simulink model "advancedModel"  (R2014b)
settings: Solver=ode45  StartTime=0.0  StopTime=1000  RelTol=1e-3

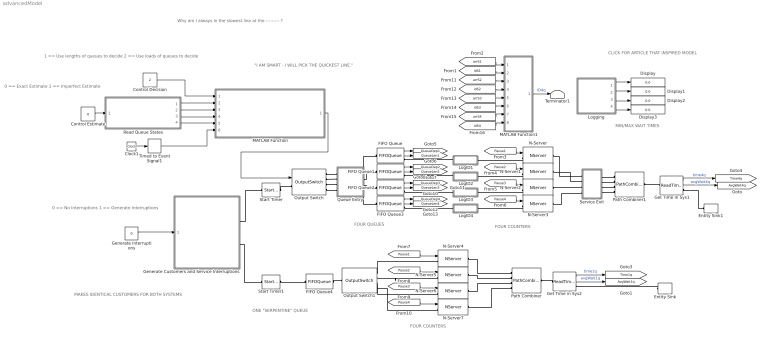
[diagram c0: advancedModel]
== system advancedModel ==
  note: 1 == Use lengths of queues to decide 2 == Use loads of queues to decide
  note: Why am I always in the slowest line at the --------- ?
  note: MAKES IDENTICAL CUSTOMERS FOR BOTH SYSTEMS
  note: "I AM SMART - I WILL PICK THE QUICKEST LINE."
  note: ONE "SERPENTINE" QUEUE
  note: FOUR COUNTERS
  note: FOUR COUNTERS
  note: FOUR QUEUES
  note: CLICK FOR ARTICLE THAT INSPIRED MODEL
  note: MIN/MAX WAIT TIMES
  note: 0 == Exact Estimate 1 == Imperfect Estimate
  note: 0 == No Interruptions 1 == Generate Interruptions
  Clock1 : Clock
  Control Decision : Constant  Value=2
  Control Estimate : Constant  Value=0
  Display{,1..3} (4 alike) : Display
  Entity Sink : EntitySink
  Entity Sink1 : EntitySink
  FIFO Queue{,1..3} (4 alike) : FIFOQueue  Capacity=inf  StatNumberDeparted=on  StatNumberInBlock=on
  FIFO Queue4 : FIFOQueue  Capacity=inf
  Generate Customers and Service Interruptions : Subsystem
  Generate Interruptions : Constant  Value=0
  Get Time In Sys1 : ReadTimer  StatTimeElapsed=on  StatAverageTimeElapsed=on
  Get Time in Sys2 : ReadTimer  TimerTag=T2  StatTimeElapsed=on  StatAverageTimeElapsed=on
  LogID1 : Subsystem
  LogID2 : Subsystem
  LogID3 : Subsystem
  LogID4 : Subsystem
  Logging : Subsystem
  MATLAB Function : MATLAB Function  TreatAsAtomicUnit=on
  MATLAB Function1 : MATLAB Function  TreatAsAtomicUnit=on
  N-Server{,1..7} (8 alike) : NServer  NumberOfServers=1  ServiceTimeFrom=Attribute  ServiceTime=sTime  AttributeName=sTime  AllowServiceControl=on
  Output Switch : OutputSwitch  NumberOutputPorts=4  SwitchingCriterion=From signal port p  InitialConditionsOpt=on
  Output Switch1 : OutputSwitch  NumberOutputPorts=4
  Path Combiner : PathCombiner  NumberInputPorts=4
  Path Combiner1 : PathCombiner  NumberInputPorts=4
  Queue Entry : Subsystem
  Read Queue States : Subsystem
  Service Exit : Subsystem
  Start Timer : StartTimer
  Start Timer1 : StartTimer  TimerTag=T2
  Terminator1 : Terminator
  Timed to Event Signal1 : TimedToEventSignal
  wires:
  Get Time In Sys1/2 -> [AvgWait4q]  "avgWait4q"
  Get Time in Sys2/2 -> [AvgWait1q]  "avgWait1q"
  [Pause1] -> N-Server/1
  [Pause2] -> N-Server1/1
  [Pause3] -> N-Server2/1
  [Pause4] -> N-Server3/1
  [Pause1] -> N-Server4/1
  [Pause2] -> N-Server5/1
  [Pause3] -> N-Server6/1
  [Pause4] -> N-Server7/1
  MATLAB Function/1(sq) -> Output Switch/1
  Get Time in Sys2/1 -> [Time1q]  "time1q"
  Get Time In Sys1/1 -> [Time4q]  "time4q"
  Logging/1(Min4q) -> Display/1
  Logging/2(Max4q) -> Display1/1
  Logging/3(Min1q) -> Display2/1
  Logging/4(Max1q) -> Display3/1
  Control Decision/1 -> MATLAB Function/1(strat)
  Generate Interruptions/1 -> Generate Customers and Service Interruptions/1(GenInterruptions)
  FIFO Queue/1 -> [QueueDep1]
  FIFO Queue/2 -> [QueueLen1]
  FIFO Queue1/1 -> [QueueDep2]
  FIFO Queue1/2 -> [QueueLen2]
  FIFO Queue2/1 -> [QueueDep3]
  FIFO Queue2/2 -> [QueueLen3]
  FIFO Queue3/1 -> [QueueDep4]
  FIFO Queue3/2 -> [QueueLen4]
  Clock1/1 -> Timed to Event Signal1/1
  Timed to Event Signal1/1 -> MATLAB Function/6(currTime)
  Read Queue States/1(queueLens) -> MATLAB Function/2(qLengths)
  Read Queue States/2(queueLoads) -> MATLAB Function/3(qLoads)
  Read Queue States/3(servStartEvents) -> MATLAB Function/4(servStartEvents)
  Read Queue States/4(servEndEvents) -> MATLAB Function/5(servEndEvents)
  [idS3] -> MATLAB Function1/6(id3)
  [idS4] -> MATLAB Function1/8(id4)
  [arrS3] -> MATLAB Function1/5(arr3)
  [idS1] -> MATLAB Function1/2(id1)
  [arrS1] -> MATLAB Function1/1(arr1)
  [arrS4] -> MATLAB Function1/7(arr4)
  [idS2] -> MATLAB Function1/4(id2)
  [arrS2] -> MATLAB Function1/3(arr2)
  MATLAB Function1/1(id) -> Terminator1/1  "ID4q"
  Control Estimate/1 -> Read Queue States/1(UnderEstimateLoad)
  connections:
  Start Timer1/RConn1 -- FIFO Queue4/LConn1
  N-Server/LConn1 -- LogID1/RConn1
  N-Server1/LConn1 -- LogID2/RConn1
  N-Server2/LConn1 -- LogID3/RConn1
  N-Server3/LConn1 -- LogID4/RConn1
  FIFO Queue4/RConn1 -- Output Switch1/LConn1
  Entity Sink/LConn1 -- Get Time in Sys2/RConn1
  Start Timer/RConn1 -- Output Switch/LConn1
  Get Time In Sys1/LConn1 -- Path Combiner1/RConn1
  Get Time in Sys2/LConn1 -- Path Combiner/RConn1
  Entity Sink1/LConn1 -- Get Time In Sys1/RConn1
  Generate Customers and Service Interruptions/RConn1 -- Start Timer/LConn1
  Generate Customers and Service Interruptions/RConn2 -- Start Timer1/LConn1
  Queue Entry/RConn1 -- FIFO Queue/LConn1
  Output Switch/RConn1 -- Queue Entry/LConn1
  Queue Entry/RConn2 -- FIFO Queue1/LConn1
  Output Switch/RConn2 -- Queue Entry/LConn2
  Output Switch/RConn3 -- Queue Entry/LConn3
  Queue Entry/RConn3 -- FIFO Queue2/LConn1
  Output Switch/RConn4 -- Queue Entry/LConn4
  Queue Entry/RConn4 -- FIFO Queue3/LConn1
  N-Server/RConn1 -- Service Exit/LConn1
  Service Exit/LConn2 -- N-Server1/RConn1
  N-Server2/RConn1 -- Service Exit/LConn3
  N-Server3/RConn1 -- Service Exit/LConn4
  Service Exit/RConn1 -- Path Combiner1/LConn1
  Service Exit/RConn2 -- Path Combiner1/LConn2
  Service Exit/RConn3 -- Path Combiner1/LConn3
  Service Exit/RConn4 -- Path Combiner1/LConn4
  Output Switch1/RConn1 -- N-Server4/LConn1
  Output Switch1/RConn2 -- N-Server5/LConn1
  Output Switch1/RConn3 -- N-Server6/LConn1
  N-Server7/LConn1 -- Output Switch1/RConn4
  N-Server4/RConn1 -- Path Combiner/LConn1
  N-Server5/RConn1 -- Path Combiner/LConn2
  N-Server6/RConn1 -- Path Combiner/LConn3
  N-Server7/RConn1 -- Path Combiner/LConn4
  LogID1/LConn1 -- FIFO Queue/RConn1
  LogID2/LConn1 -- FIFO Queue1/RConn1
  LogID3/LConn1 -- FIFO Queue2/RConn1
  LogID4/LConn1 -- FIFO Queue3/RConn1

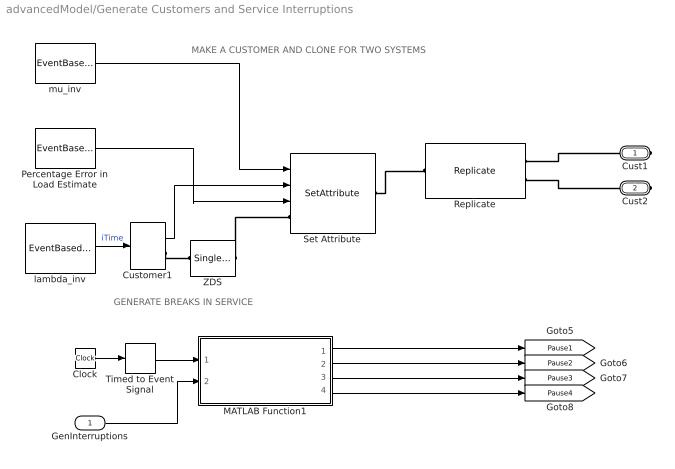
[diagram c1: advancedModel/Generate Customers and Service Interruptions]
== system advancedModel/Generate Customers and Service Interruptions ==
  note: MAKE A CUSTOMER AND CLONE FOR TWO SYSTEMS
  note: GENERATE BREAKS IN SERVICE
  GenInterruptions : Inport
  Clock : Clock
  Customer1 : TimeBasedEntityGenerator  GenerateEntitiesUpon=Intergeneration time from port t  Distribution=Exponential  InitialSeed=35250  Mean=0.9  GenerateEntityAtSimulationStart=off  StatNumberDeparted=on
  MATLAB Function1 : MATLAB Function  TreatAsAtomicUnit=on
  Percentage Error in Load Estimate : EventBasedRandomNumber  Distribution=Uniform  meanExp=2  minUnif=-100  maxUnif=0  Seed=22753
  Replicate : Replicate  NumberOutputPorts=2
  Set Attribute : SetAttribute  AttributeName=sTime|ID|estErrPerc  AttributeFrom=Signal port|Signal port|Signal port  AttributeValue=1|1|1  AttributeTreatAsVector=1|1|1  EvaluatedAttributeValue={ [];[];[]}
  Timed to Event Signal : TimedToEventSignal
  ZDS : SingleServer  ServiceTime=0  AttributeName=sTime
  lambda_inv : EventBasedRandomNumber  meanExp=0.7  Seed=35250
  mu_inv : EventBasedRandomNumber  meanExp=2  Seed=25970
  Cust1 : PMIOPort  Port=1  Side=Right
  Cust2 : PMIOPort  Port=2  Side=Right
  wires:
  mu_inv/1 -> Set Attribute/1
  Customer1/1 -> Set Attribute/2
  Clock/1 -> Timed to Event Signal/1
  MATLAB Function1/1(pause1) -> [Pause1]
  MATLAB Function1/2(pause2) -> [Pause2]
  MATLAB Function1/3(pause3) -> [Pause3]
  MATLAB Function1/4(pause4) -> [Pause4]
  Timed to Event Signal/1 -> MATLAB Function1/1(currTime)
  GenInterruptions/1 -> MATLAB Function1/2(genInt)
  Percentage Error in Load Estimate/1 -> Set Attribute/3
  lambda_inv/1 -> Customer1/1  "iTime"
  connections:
  Replicate/RConn1 -- Cust1/RConn1
  Customer1/RConn1 -- ZDS/LConn1
  Replicate/RConn2 -- Cust2/RConn1
  ZDS/RConn1 -- Set Attribute/LConn1
  Set Attribute/RConn1 -- Replicate/LConn1

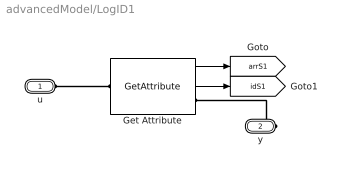
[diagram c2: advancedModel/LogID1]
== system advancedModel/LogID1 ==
  Get Attribute : GetAttribute  AttributeName=ID  StatNumberDeparted=on  EvaluatedDefaultAttributeValue={ []}
  u : PMIOPort  Port=1  Side=Left
  y : PMIOPort  Port=2  Side=Right
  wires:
  Get Attribute/1 -> [arrS1]
  Get Attribute/2 -> [idS1]
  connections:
  y/RConn1 -- Get Attribute/RConn1
  Get Attribute/LConn1 -- u/RConn1

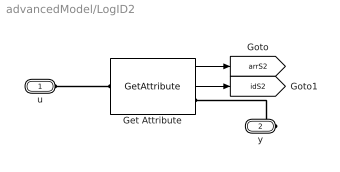
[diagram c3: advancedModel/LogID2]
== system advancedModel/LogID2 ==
  Get Attribute : GetAttribute  AttributeName=ID  StatNumberDeparted=on  EvaluatedDefaultAttributeValue={ []}
  u : PMIOPort  Port=1  Side=Left
  y : PMIOPort  Port=2  Side=Right
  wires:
  Get Attribute/1 -> [arrS2]
  Get Attribute/2 -> [idS2]
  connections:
  y/RConn1 -- Get Attribute/RConn1
  Get Attribute/LConn1 -- u/RConn1

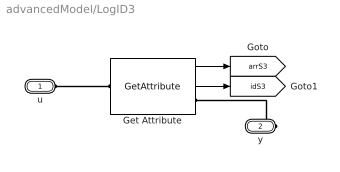
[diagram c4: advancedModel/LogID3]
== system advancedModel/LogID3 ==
  Get Attribute : GetAttribute  AttributeName=ID  StatNumberDeparted=on  EvaluatedDefaultAttributeValue={ []}
  u : PMIOPort  Port=1  Side=Left
  y : PMIOPort  Port=2  Side=Right
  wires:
  Get Attribute/1 -> [arrS3]
  Get Attribute/2 -> [idS3]
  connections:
  y/RConn1 -- Get Attribute/RConn1
  Get Attribute/LConn1 -- u/RConn1

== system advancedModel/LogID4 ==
  Get Attribute : GetAttribute  AttributeName=ID  StatNumberDeparted=on  EvaluatedDefaultAttributeValue={ []}
  u : PMIOPort  Port=1  Side=Left
  y : PMIOPort  Port=2  Side=Right
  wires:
  Get Attribute/1 -> [arrS4]
  Get Attribute/2 -> [idS4]
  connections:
  y/RConn1 -- Get Attribute/RConn1
  Get Attribute/LConn1 -- u/RConn1

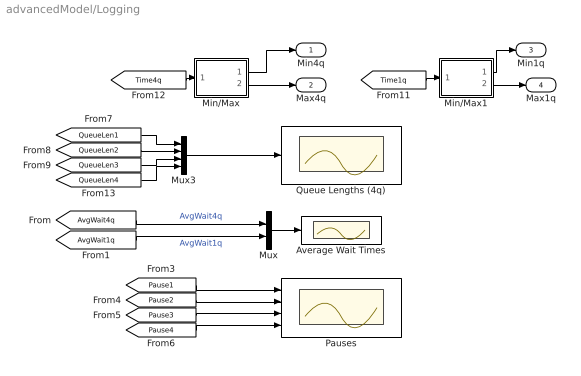
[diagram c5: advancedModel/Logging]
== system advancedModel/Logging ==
  Average Wait Times : Scope
  Min/Max : Subsystem  TreatAsAtomicUnit=on
  Min/Max1 : Subsystem  TreatAsAtomicUnit=on
  Mux : Mux  Inputs=2
  Mux3 : Mux
  Pauses : Scope  NumInputPorts=4
  Queue Lengths (4q) : Scope
  Min4q : Outport
  Max4q : Outport  Port=2
  Min1q : Outport  Port=3
  Max1q : Outport  Port=4
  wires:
  Min/Max/1(min) -> Min4q/1
  Min/Max/2(max) -> Max4q/1
  Min/Max1/1(min) -> Min1q/1
  Min/Max1/2(max) -> Max1q/1
  [Time4q] -> Min/Max/1(u)
  [Time1q] -> Min/Max1/1(u)
  Mux/1 -> Average Wait Times/1
  [AvgWait4q] -> Mux/1  "AvgWait4q"
  [AvgWait1q] -> Mux/2  "AvgWait1q"
  Mux3/1 -> Queue Lengths (4q)/1
  [Pause2] -> Pauses/2
  [Pause1] -> Pauses/1
  [Pause3] -> Pauses/3
  [Pause4] -> Pauses/4
  [QueueLen2] -> Mux3/2
  [QueueLen3] -> Mux3/3
  [QueueLen1] -> Mux3/1
  [QueueLen4] -> Mux3/4

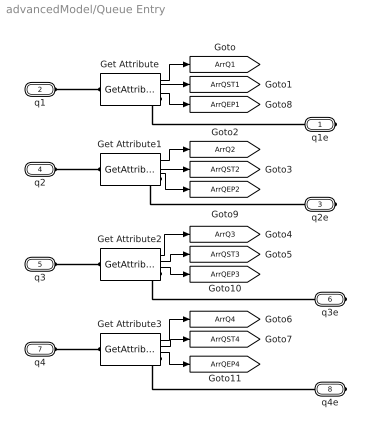
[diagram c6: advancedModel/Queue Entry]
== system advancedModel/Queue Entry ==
  Get Attribute{,1..3} (4 alike) : GetAttribute  AttributeName=sTime|estErrPerc  AttributeMissing=Error|Error  AttributeDefaultValue=1|1  AttributeTreatAsVector=1|1  AttributeSendTiming=After entity departure|After entity departure  StatNumberDeparted=on  EvaluatedDefaultAttributeValue={ [];[]}
  q1e : PMIOPort  Port=1  Side=Right
  q1 : PMIOPort  Port=2  Side=Left
  q2e : PMIOPort  Port=3  Side=Right
  q2 : PMIOPort  Port=4  Side=Left
  q3 : PMIOPort  Port=5  Side=Left
  q3e : PMIOPort  Port=6  Side=Right
  q4 : PMIOPort  Port=7  Side=Left
  q4e : PMIOPort  Port=8  Side=Right
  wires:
  Get Attribute3/1 -> [ArrQ4]
  Get Attribute3/2 -> [ArrQST4]
  Get Attribute1/2 -> [ArrQST2]
  Get Attribute1/1 -> [ArrQ2]
  Get Attribute/2 -> [ArrQST1]
  Get Attribute2/1 -> [ArrQ3]
  Get Attribute2/2 -> [ArrQST3]
  Get Attribute/1 -> [ArrQ1]
  Get Attribute/3 -> [ArrQEP1]
  Get Attribute1/3 -> [ArrQEP2]
  Get Attribute2/3 -> [ArrQEP3]
  Get Attribute3/3 -> [ArrQEP4]
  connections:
  Get Attribute1/RConn1 -- q2e/RConn1
  q4/RConn1 -- Get Attribute3/LConn1
  q3/RConn1 -- Get Attribute2/LConn1
  q2/RConn1 -- Get Attribute1/LConn1
  Get Attribute3/RConn1 -- q4e/RConn1
  Get Attribute2/RConn1 -- q3e/RConn1
  Get Attribute/RConn1 -- q1e/RConn1
  q1/RConn1 -- Get Attribute/LConn1

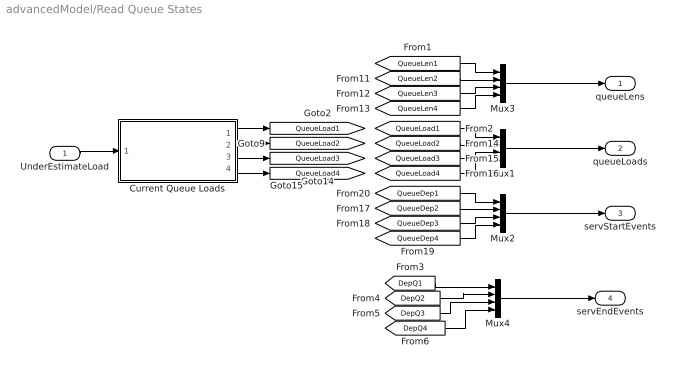
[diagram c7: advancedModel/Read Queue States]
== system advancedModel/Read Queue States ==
  UnderEstimateLoad : Inport
  Current Queue Loads : Subsystem
  Mux{1..4} (4 alike) : Mux
  queueLens : Outport
  queueLoads : Outport  Port=2
  servStartEvents : Outport  Port=3
  servEndEvents : Outport  Port=4
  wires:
  [QueueLen2] -> Mux3/2
  [QueueLen3] -> Mux3/3
  [QueueLen1] -> Mux3/1
  [QueueLen4] -> Mux3/4
  Current Queue Loads/1(ql1) -> [QueueLoad1]
  Current Queue Loads/2(ql2) -> [QueueLoad2]
  Current Queue Loads/3(ql3) -> [QueueLoad3]
  Current Queue Loads/4(ql4) -> [QueueLoad4]
  [QueueLoad2] -> Mux1/2
  [QueueLoad3] -> Mux1/3
  [QueueLoad1] -> Mux1/1
  [QueueLoad4] -> Mux1/4
  Mux2/1 -> servStartEvents/1
  [QueueDep2] -> Mux2/2
  [QueueDep3] -> Mux2/3
  [QueueDep1] -> Mux2/1
  [QueueDep4] -> Mux2/4
  Mux3/1 -> queueLens/1
  Mux1/1 -> queueLoads/1
  [DepQ2] -> Mux4/2
  [DepQ1] -> Mux4/1
  [DepQ4] -> Mux4/4
  [DepQ3] -> Mux4/3
  Mux4/1 -> servEndEvents/1
  UnderEstimateLoad/1 -> Current Queue Loads/1(UnderEstimateLoad)

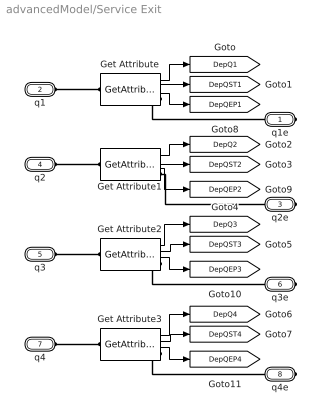
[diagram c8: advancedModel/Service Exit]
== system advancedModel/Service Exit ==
  Get Attribute{,1..3} (4 alike) : GetAttribute  AttributeName=sTime|estErrPerc  AttributeMissing=Error|Error  AttributeDefaultValue=1|1  AttributeTreatAsVector=1|1  AttributeSendTiming=After entity departure|After entity departure  StatNumberDeparted=on  EvaluatedDefaultAttributeValue={ [];[]}
  q1e : PMIOPort  Port=1  Side=Right
  q1 : PMIOPort  Port=2  Side=Left
  q2e : PMIOPort  Port=3  Side=Right
  q2 : PMIOPort  Port=4  Side=Left
  q3 : PMIOPort  Port=5  Side=Left
  q3e : PMIOPort  Port=6  Side=Right
  q4 : PMIOPort  Port=7  Side=Left
  q4e : PMIOPort  Port=8  Side=Right
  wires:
  Get Attribute/1 -> [DepQ1]
  Get Attribute2/2 -> [DepQST3]
  Get Attribute2/1 -> [DepQ3]
  Get Attribute/2 -> [DepQST1]
  Get Attribute1/1 -> [DepQ2]
  Get Attribute1/2 -> [DepQST2]
  Get Attribute3/2 -> [DepQST4]
  Get Attribute3/1 -> [DepQ4]
  Get Attribute/3 -> [DepQEP1]
  Get Attribute1/3 -> [DepQEP2]
  Get Attribute2/3 -> [DepQEP3]
  Get Attribute3/3 -> [DepQEP4]
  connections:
  q1/RConn1 -- Get Attribute/LConn1
  Get Attribute/RConn1 -- q1e/RConn1
  Get Attribute2/RConn1 -- q3e/RConn1
  Get Attribute3/RConn1 -- q4e/RConn1
  q2/RConn1 -- Get Attribute1/LConn1
  q3/RConn1 -- Get Attribute2/LConn1
  q4/RConn1 -- Get Attribute3/LConn1
  Get Attribute1/RConn1 -- q2e/RConn1

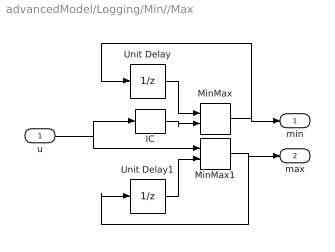
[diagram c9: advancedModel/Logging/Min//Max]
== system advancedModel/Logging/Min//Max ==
  u : Inport
  IC : InitialCondition  Value=100
  MinMax : MinMax  Inputs=2
  MinMax1 : MinMax  Function=max  Inputs=2
  Unit Delay : UnitDelay  InitialCondition=100  SampleTime=-1
  Unit Delay1 : UnitDelay  SampleTime=-1
  min : Outport
  max : Outport  Port=2
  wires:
  Unit Delay1/1 -> MinMax1/2
  MinMax1/1 -> Unit Delay1/1, max/1
  Unit Delay/1 -> MinMax/1
  MinMax/1 -> Unit Delay/1, min/1
  u/1 -> MinMax1/1, IC/1
  IC/1 -> MinMax/2

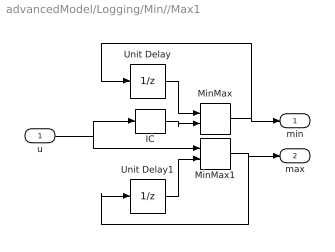
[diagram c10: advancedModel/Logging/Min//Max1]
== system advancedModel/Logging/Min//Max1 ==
  u : Inport
  IC : InitialCondition  Value=100
  MinMax : MinMax  Inputs=2
  MinMax1 : MinMax  Function=max  Inputs=2
  Unit Delay : UnitDelay  InitialCondition=100  SampleTime=-1
  Unit Delay1 : UnitDelay  SampleTime=-1
  min : Outport
  max : Outport  Port=2
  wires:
  IC/1 -> MinMax/2
  u/1 -> IC/1, MinMax1/1
  MinMax/1 -> min/1, Unit Delay/1
  Unit Delay/1 -> MinMax/1
  MinMax1/1 -> max/1, Unit Delay1/1
  Unit Delay1/1 -> MinMax1/2

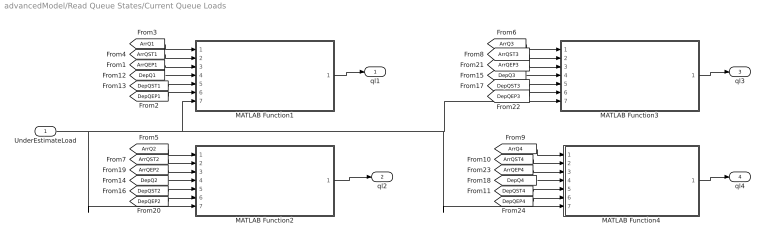
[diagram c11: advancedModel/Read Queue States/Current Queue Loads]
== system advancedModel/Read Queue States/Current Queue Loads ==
  UnderEstimateLoad : Inport
  MATLAB Function1 : MATLAB Function  TreatAsAtomicUnit=on
  MATLAB Function2 : MATLAB Function  TreatAsAtomicUnit=on
  MATLAB Function3 : MATLAB Function  TreatAsAtomicUnit=on
  MATLAB Function4 : MATLAB Function  TreatAsAtomicUnit=on
  ql1 : Outport
  ql2 : Outport  Port=2
  ql3 : Outport  Port=3
  ql4 : Outport  Port=4
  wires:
  [DepQST1] -> MATLAB Function1/5(depSTime)
  [ArrQ1] -> MATLAB Function1/1(arrEvent)
  [ArrQST1] -> MATLAB Function1/2(arrSTime)
  [DepQ1] -> MATLAB Function1/4(depEvent)
  [ArrQST2] -> MATLAB Function2/2(arrSTime)
  [ArrQ2] -> MATLAB Function2/1(arrEvent)
  [DepQ2] -> MATLAB Function2/4(depEvent)
  [DepQST2] -> MATLAB Function2/5(depSTime)
  MATLAB Function1/1(qSTime) -> ql1/1
  [DepQEP1] -> MATLAB Function1/6(depEP)
  [ArrQEP1] -> MATLAB Function1/3(arrEP)
  [ArrQEP2] -> MATLAB Function2/3(arrEP)
  [DepQEP2] -> MATLAB Function2/6(depEP)
  MATLAB Function2/1(qSTime) -> ql2/1
  [DepQST3] -> MATLAB Function3/5(depSTime)
  [ArrQST3] -> MATLAB Function3/2(arrSTime)
  [ArrQEP3] -> MATLAB Function3/3(arrEP)
  [DepQ3] -> MATLAB Function3/4(depEvent)
  [ArrQ3] -> MATLAB Function3/1(arrEvent)
  [DepQEP3] -> MATLAB Function3/6(depEP)
  [DepQ4] -> MATLAB Function4/4(depEvent)
  [ArrQ4] -> MATLAB Function4/1(arrEvent)
  [ArrQST4] -> MATLAB Function4/2(arrSTime)
  [DepQST4] -> MATLAB Function4/5(depSTime)
  [DepQEP4] -> MATLAB Function4/6(depEP)
  [ArrQEP4] -> MATLAB Function4/3(arrEP)
  MATLAB Function3/1(qSTime) -> ql3/1
  MATLAB Function4/1(qSTime) -> ql4/1
  UnderEstimateLoad/1 -> MATLAB Function2/7(uEst), MATLAB Function4/7(uEst), MATLAB Function3/7(uEst), MATLAB Function1/7(uEst)

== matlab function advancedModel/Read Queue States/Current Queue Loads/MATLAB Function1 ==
function qSTime = currentQueueLoad(arrEvent,arrSTime,arrEP,depEvent,depSTime,depEP,uEst)
%#codegen
persistent arrEventCount depEventCount qSTimeSum

if isempty(arrEventCount)
    arrEventCount = 0;
end
if isempty(depEventCount)
    depEventCount = 0;
end
if isempty(qSTimeSum)
    qSTimeSum = 0;
end

if arrEventCount ~= arrEvent
    % Arrival into queue
    arrEventCount = arrEvent;
    qSTimeSum = qSTimeSum + (arrSTime + (uEst*arrSTime*arrEP/100));
elseif depEventCount ~= depEvent
    % Departure into server
    depEventCount = depEvent;
    qSTimeSum = qSTimeSum - (depSTime + (uEst*depSTime*depEP/100));
end
qSTime = qSTimeSum;

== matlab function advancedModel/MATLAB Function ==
function sq = bestQueueEstimate(strat,qLengths,qLoads,servStartEvents,servEndEvents,currTime)
%#codegen
persistent servStartEventsSt servStartTimes servEndEventsSt

if isempty(servStartEventsSt)
    servStartEventsSt = zeros(4,1);
end

if isempty(servEndEventsSt)
    servEndEventsSt = zeros(4,1);
end

if isempty(servStartTimes)
    servStartTimes = -ones(4,1);
end

if strat ~= 1
    % Update time adjustments for service
    if nnz(servStartEvents ~= servStartEventsSt) ~= 0
        for k = 1:4
            if servStartEvents(k) ~= servStartEventsSt(k)
                servStartTimes(k) = currTime;
            end
        end
        servStartEventsSt = servStartEvents;
    end
    if nnz(servEndEvents ~= servEndEventsSt) ~= 0
        for k = 1:4
            if servEndEvents(k) ~= servEndEventsSt(k)
                servStartTimes(k) = -1;
            end
        end
        servEndEventsSt = servEndEvents;
    end
end

if strat == 1
    % Pick a short queue at random
    minVal = min(qLengths);
    minIdx = find(qLengths == minVal);
    randSel = randi([1 length(minIdx)]);
    sq = minIdx(randSel);
else 
    % Pick the least loaded queue
    qL = qLoads;
    for k = 1:4
        if servStartTimes(k) > 0
            qL(k) = qL(k) - (currTime-servStartTimes(k));
        end
    end
    minVal = min(qL);
    minIdx = find(qL == minVal);
    randSel = randi([1 length(minIdx)]);
    sq = minIdx(randSel);
end

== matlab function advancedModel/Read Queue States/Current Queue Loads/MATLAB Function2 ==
function qSTime = currentQueueLoad(arrEvent,arrSTime,arrEP,depEvent,depSTime,depEP,uEst)
%#codegen
persistent arrEventCount depEventCount qSTimeSum

if isempty(arrEventCount)
    arrEventCount = 0;
end
if isempty(depEventCount)
    depEventCount = 0;
end
if isempty(qSTimeSum)
    qSTimeSum = 0;
end

if arrEventCount ~= arrEvent
    % Arrival into queue
    arrEventCount = arrEvent;
    qSTimeSum = qSTimeSum + (arrSTime + (uEst*arrSTime*arrEP/100));
elseif depEventCount ~= depEvent
    % Departure into server
    depEventCount = depEvent;
    qSTimeSum = qSTimeSum - (depSTime + (uEst*depSTime*depEP/100));
end
qSTime = qSTimeSum;

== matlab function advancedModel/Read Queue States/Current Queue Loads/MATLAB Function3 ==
function qSTime = currentQueueLoad(arrEvent,arrSTime,arrEP,depEvent,depSTime,depEP,uEst)
%#codegen
persistent arrEventCount depEventCount qSTimeSum

if isempty(arrEventCount)
    arrEventCount = 0;
end
if isempty(depEventCount)
    depEventCount = 0;
end
if isempty(qSTimeSum)
    qSTimeSum = 0;
end

if arrEventCount ~= arrEvent
    % Arrival into queue
    arrEventCount = arrEvent;
    qSTimeSum = qSTimeSum + (arrSTime + (uEst*arrSTime*arrEP/100));
elseif depEventCount ~= depEvent
    % Departure into server
    depEventCount = depEvent;
    qSTimeSum = qSTimeSum - (depSTime + (uEst*depSTime*depEP/100));
end
qSTime = qSTimeSum;

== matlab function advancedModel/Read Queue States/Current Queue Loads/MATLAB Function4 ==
function qSTime = currentQueueLoad(arrEvent,arrSTime,arrEP,depEvent,depSTime,depEP,uEst)
%#codegen
persistent arrEventCount depEventCount qSTimeSum

if isempty(arrEventCount)
    arrEventCount = 0;
end
if isempty(depEventCount)
    depEventCount = 0;
end
if isempty(qSTimeSum)
    qSTimeSum = 0;
end

if arrEventCount ~= arrEvent
    % Arrival into queue
    arrEventCount = arrEvent;
    qSTimeSum = qSTimeSum + (arrSTime + (uEst*arrSTime*arrEP/100));
elseif depEventCount ~= depEvent
    % Departure into server
    depEventCount = depEvent;
    qSTimeSum = qSTimeSum - (depSTime + (uEst*depSTime*depEP/100));
end
qSTime = qSTimeSum;

== matlab function advancedModel/Generate Customers and
Service Interruptions/MATLAB Function1 ==
 function [pause1,pause2,pause3,pause4] = genPause(currTime,genInt)
%#codegen

    persistent nextPause1 nextPause2 nextPause3 nextPause4

    if isempty(nextPause1)
        nextPause1 = [0 0];
    end
    if isempty(nextPause2)
        nextPause2 = [0 0];
    end
    if isempty(nextPause3)
        nextPause3 = [0 0];
    end
    if isempty(nextPause4)
        nextPause4 = [0 0];
    end
    if genInt > 0
        if nextPause1(1) == 0
            nextPause1 = genNextPauseVals(currTime);
            nextPause2 = genNextPauseVals(currTime);
            nextPause3 = genNextPauseVals(currTime);
            nextPause4 = genNextPauseVals(currTime);
        end

        [pause1, nextPause1] = locGenPause(currTime, nextPause1);
        [pause2, nextPause2] = locGenPause(currTime, nextPause2);
        [pause3, nextPause3] = locGenPause(currTime, nextPause3);
        [pause4, nextPause4] = locGenPause(currTime, nextPause4);
    else
        pause1 = 0;
        pause2 = 0;
        pause3 = 0;
        pause4 = 0;
    end
end

function [pVal, nP] = locGenPause(cT, nP)
    if cT >= nP(1)
        if cT < nP(1) + nP(2)
            pVal = 1;
        else
            pVal = 0;
            nP = genNextPauseVals(cT);
        end
    else
        pVal = 0;
    end
end

function nP = genNextPauseVals(cT)
    nP = [0 0];
    nP(1) = cT + (10+exprnd(5));
    nP(2) = 2 + rand(1)*2;
end

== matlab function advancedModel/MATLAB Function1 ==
function id = idMerge(arr1,id1,arr2,id2,arr3,id3,arr4,id4)
%#codegen
persistent arr1S arr2S arr3S arr4S

if isempty(arr1S)
    arr1S = 1;
end
if isempty(arr2S)
    arr2S = 1;
end
if isempty(arr3S)
    arr3S = 1;
end
if isempty(arr4S)
    arr4S = 1;
end
id = 0;
if arr1 ~= arr1S
    id = id1;
    arr1S = arr1;
elseif arr2 ~= arr2S
    id = id2;
    arr2S = arr2;
elseif arr3 ~= arr3S
    id = id3;
    arr3S = arr3;
elseif arr4 ~= arr4S
    id = id4;
    arr4S = arr4;
end
